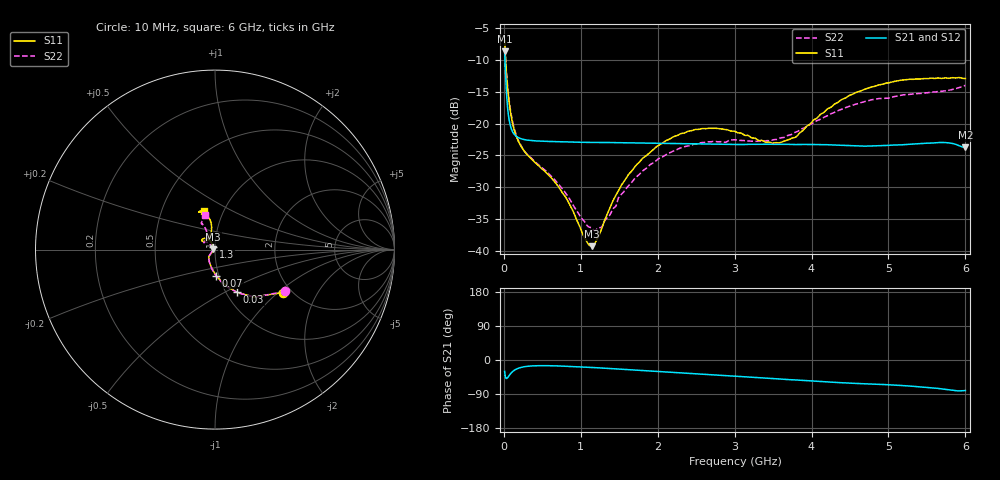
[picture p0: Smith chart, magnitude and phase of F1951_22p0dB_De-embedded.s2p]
! Integrated Device Technology
! Corporate Headquarters
! 6024 Silver Creek Valley Road
! San Jose, CA 95138  USA
! Phone:  1-408-284-8200
! Toll Free:  1-800-223-1366
! Webpage:  http://www.idt.com/
! Timing and RF Division
! 515 Groton Road, Suite 102
! Westford, MA 01886-6024
! Device:  F1951
! Description: 6-bit 0.5 dB Digital Step Attenuator
! Frequency:  100.0 -  4000.00 MHz
! Package:  4x4 mm Thin QFN Plastic Package: 24 pin
! Ports:  2 RF, 6 DC
!  Pin  1  = NC
!  Pin  2  = RF1  =  Port 1
!  Pin  3  = GND
!  Pin  4  = NC
!  Pin  5  = Serial Data Out (SDO)
!  Pin  6  = NC
!  Pin  7  = Reset Bar ( RSTb)
!  Pin  8  = Clock (CLK)
!  Pin  9  = Chip Select Bar (CSb)
!  Pin 10  = NC
!  Pin 11  = Serial Data In (SDI)
!  Pin 12  = NC
!  Pin 13  = NC
!  Pin 14  = VDD
!  Pin 15  = NC
!  Pin 16  = GND
!  Pin 17  = RF2  =  Port 2
!  Pin 18  = NC
!  Pin 19  = GND
!  Pin 20  = GND
!  Pin 21  = GND
!  Pin 22  = GND
!  Pin 23  = GND
!  Pin 24  = GND
! State:  44
! Atten State:  22.0 dB
! Voltage:  +3.30 Volts
! Current:  0.478 mA
! Data:  The device was measured on a F195X evaluation board which has
!  individual transmission lines to the RF pins.  Data was collected
!  de-embedded using a Automatic Fixture Removal [AFR] (Keysight Technologies).
!  The reference plane is the edge of the package pin.
! Misc:  Lot Code  1225BCA
!  Action Tracker AT0399
! Date Measured:  2018-09-13
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# GHz S dB R 50
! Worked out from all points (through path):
!   600 points, 10 MHz to 6 GHz, reference 50 ohm
!   highest |S21| = -8.63 dB at 10 MHz (marker M1); lowest = -23.8 dB at 6 GHz (marker M2)
!   group delay of S21, straight-line fit = 30.7 ps
!   lowest |S11| = -39.3 dB at 1.14 GHz (marker M3), VSWR 1.02, Z = 48.9 + j0.188 ohm
!   |S11| at or under -10 dB: 23 MHz to end of sweep
!   |S22| runs from -36.8 to -6.9 dB; largest |S21 - S12| = 0.00021
!   S11 on the Smith chart (normalised r, x): 10 MHz: 1.81, -1.08; 30 MHz: 1.12, -0.58; 70 MHz: 0.97, -0.29; 1.3 GHz: 0.98, +0.03; 6 GHz: 0.80, +0.37
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0.01  -6.96 -32.2  -8.63 -30.0  -8.63 -30.0  -6.90 -31.0
0.03  -11.45 -62.7  -14.19 -48.8  -14.19 -48.9  -11.17 -61.5
0.07  -16.77 -87.2  -19.49 -40.8  -19.49 -40.8  -16.49 -86.7
0.14  -21.20 -108.0  -21.75 -26.6  -21.75 -26.6  -20.99 -107.1
0.24  -23.88 -122.2  -22.44 -18.8  -22.44 -18.8  -23.81 -121.7
0.71  -29.92 -134.0  -22.85 -15.7  -22.84 -15.8  -29.53 -137.0
1.01  -36.93 -153.0  -22.94 -18.4  -22.94 -18.4  -34.91 -150.8
1.14  -39.30 169.8  -22.96 -19.7  -22.95 -19.6  -36.42 -170.3
1.21  -38.26 146.6  -22.96 -20.4  -22.96 -20.4  -36.57 174.6
1.3  -35.56 127.5  -22.97 -21.5  -22.97 -21.5  -35.63 156.7
1.43  -31.87 118.0  -23.00 -23.1  -23.00 -23.1  -33.28 142.9
1.61  -28.20 115.6  -23.02 -25.2  -23.02 -25.3  -29.93 133.6
2.01  -23.43 123.8  -23.10 -30.5  -23.10 -30.5  -25.54 134.9
2.49  -20.91 136.8  -23.20 -36.6  -23.19 -36.6  -23.20 142.4
3.01  -21.25 146.9  -23.28 -43.1  -23.28 -43.0  -22.54 146.1
3.58  -23.03 125.8  -23.25 -50.1  -23.25 -50.1  -22.33 128.9
3.79  -22.15 110.1  -23.30 -52.7  -23.30 -52.7  -21.35 121.9
4.01  -19.66 101.4  -23.29 -55.4  -23.29 -55.4  -19.99 116.5
4.49  -15.57 99.3  -23.46 -61.1  -23.46 -61.0  -17.28 114.7
5.01  -13.55 108.0  -23.41 -65.4  -23.41 -65.4  -15.97 117.4
5.72  -12.82 112.6  -22.97 -77.0  -22.96 -77.0  -14.84 110.5
6  -12.89 106.3  -23.76 -80.4  -23.75 -80.4  -13.97 106.6
